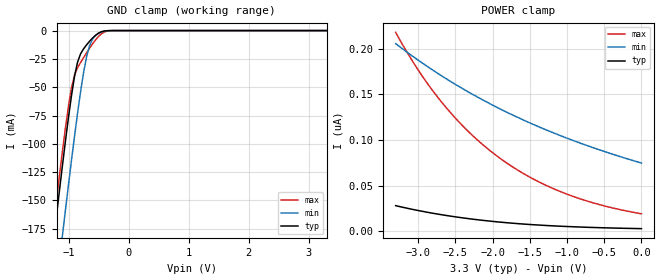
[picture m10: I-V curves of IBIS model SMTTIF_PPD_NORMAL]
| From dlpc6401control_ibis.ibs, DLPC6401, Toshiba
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[Model]   SMTTIF_PPD_NORMAL
Model_type   Input
Polarity   Non-Inverting
Vinl =   0.8000V
Vinh =   2.0000V
C_comp   1.423pF   NA   NA
|Variable   typ   min   max
[Voltage range]  3.3   3.0   3.6
[Temperature Range]   25.0000   125.000   0.000
[POWER Clamp Reference]   3.3000V   3.0000V   3.6000V
[GND Clamp Reference]   0.000V   0.000V   0.000V
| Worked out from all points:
|   GND clamp passes 1 mA (typ) near -0.45 V on its own axis
[GND_clamp]
| voltage   I(typ)   I(min)   I(max)
-3.3V     -1.18A     -1.24A     -1.166A
-1.3V     -209.3mA   -272.3mA   -195.2mA
-1.25V    -186.1mA   -249mA     -172.2mA
-1.2V     -163.2mA   -225.9mA   -149.6mA
-1.1V     -118.5mA   -180.3mA   -105.8mA
-950mV    -57.05mA   -114.1mA   -50.29mA
-850mV    -27.88mA   -73.01mA   -32.78mA
-700mV    -12.61mA   -23.19mA   -19.66mA
-600mV    -6.597mA   -7.45mA    -11.71mA
-500mV    -2.24mA    -2.388mA   -5.154mA
-300mV    -17.81uA   -59.37uA   -84.02uA
3.3V      3.035nA    82.23nA    15.46nA
[POWER_clamp]
| voltage   I(typ)   I(min)   I(max)
-3.3V     28.21nA    205.5nA    217.8nA
-3.15V    25.46nA    196.3nA    196.4nA
-3V       22.94nA    187.5nA    176.9nA
-2.85V    20.61nA    179.1nA    159.2nA
-2.65V    17.84nA    168.5nA    138.2nA
-2.3V     13.79nA    151.5nA    107.4nA
-2.1V     11.86nA    142.6nA    92.84nA
-1.9V     10.22nA    134.2nA    80.12nA
-1.5V     7.605nA    118.8nA    59.45nA
-1.05V    5.565nA    103.6nA    42.36nA
-550mV    4.092nA    88.89nA    29.07nA
0V        3.04nA     74.83nA    19.29nA
